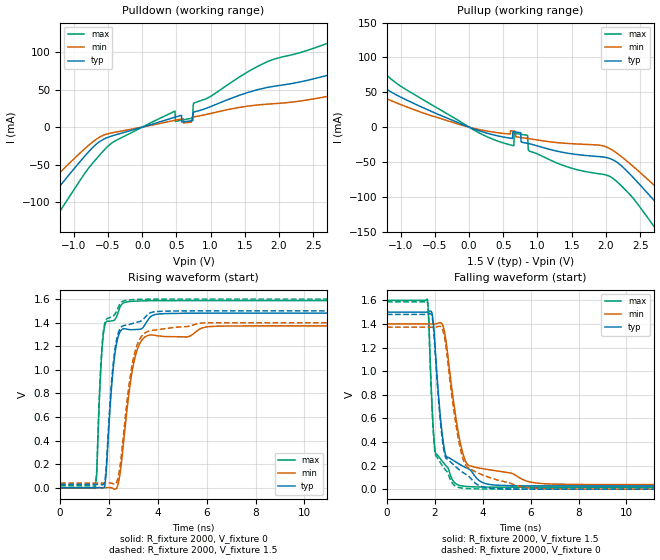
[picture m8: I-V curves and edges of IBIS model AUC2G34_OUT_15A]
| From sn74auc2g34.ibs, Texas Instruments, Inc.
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[Model]   AUC2G34_OUT_15A
Model_type  Output
Vref =   0
Rref =   2000
Cref =   15p
Vmeas =   0.75
| variable   typ   min   max
C_comp   6.42pF   1.69pF   19.07pF
| C_pullup   6.14pF   1.69pF   19.07pF
| C_pulldown   6.71pF   3.61pF   15.24pF
[Temperature Range]   40   100   -40
| Ambient temperature   25   85   -40
[Voltage range]   1.5   1.4   1.6
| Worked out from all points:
|   slope of the pulldown table from 0 to 0.225 V, typ, clamps not added: 36.6 ohm
|   slope of the pullup table from 0 to 0.225 V, typ, clamps not added: 29.5 ohm
|   rising waveform, R_fixture 2000, V_fixture 0: 20-80 % time 344ps typ, 515ps min, 222ps max; typ from 0 V to 1.48 V
|   falling waveform, R_fixture 2000, V_fixture 1.5: 20-80 % time 403ps typ, 614ps min, 233ps max; typ from 1.5 V to 0.027 V
|   rising waveform, R_fixture 2000, V_fixture 1.5: 20-80 % time 338ps typ, 508ps min, 219ps max; typ from 0.027 V to 1.5 V
|   falling waveform, R_fixture 2000, V_fixture 0: 20-80 % time 406ps typ, 619ps min, 231ps max; typ from 1.48 V to 0 V
[Pulldown]
| AUC2G34_OUT_15A
|   Voltage   I(typ)   I(min)   I(max)
-3.6V     -343.5mA   -285.3mA   -424.2mA
-2.1V     -178.7mA   -143.8mA   -232mA
-1.795V   -144.9mA   -115.3mA   -192.2mA
-1.395V   -99.99mA   -78.12mA   -138.8mA
-395mV    -10.45mA   -6.753mA   -18.28mA
480mV     13.33mA    9.224mA    21.44mA
485mV     13.46mA    9.315mA    7.619mA
735mV     8.725mA    13.4mA     12.06mA
755mV     20.22mA    13.7mA     32.02mA
1.69V     50.1mA     29.63mA    81.31mA
3.34V     86.08mA    49.98mA    134.3mA
7.2V      80.61mA    45.5mA     141.2mA
[Pullup]
| AUC2G34_OUT_15A
|   Voltage   I(typ)   I(min)   I(max)
-3.6V     253.3mA    194.5mA    303.7mA
-2.87V    186.5mA    147.2mA    232.6mA
-2.45V    149.4mA    116mA      191.5mA
-1.91V    104.2mA    79.12mA    139.3mA
100mV     -3.652mA   -2.395mA   -5.808mA
650mV     -6.722mA   -5.655mA   -26.6mA
855mV     -23.23mA   -16.19mA   -11.7mA
885mV     -23.9mA    -16.64mA   -34.51mA
2.105V    -46.98mA   -33.57mA   -73.64mA
2.765V    -111.9mA   -88.75mA   -150.9mA
3.365V    -178.9mA   -144.3mA   -231.8mA
7.2V      -606.7mA   -511.1mA   -734.8mA
[Ramp]
| AUC2G34_OUT_15A
| variable   typ   min   max
dV/dt_r   0.89/3.46E-10   0.83/5.21E-10   0.96/2.24E-10
dV/dt_f   0.89/4.05E-10   0.82/6.15E-10   0.96/2.36E-10
R_load = 2000
[Rising Waveform]
| AUC2G34_OUT_15A
R_fixture =   2000
C_fixture =   0
L_fixture =   0
V_fixture =   0
V_fixture_min = 0
V_fixture_max = 0
|   Time   V(typ)   V(min)   V(max)
0s        7.019nV    26.23nV    876.1pV
1.43ns    -7.447uV   -3.74uV    -6.582mV
1.495ns   52.17uV    -6.646uV   114.3mV
1.68ns    -986.3uV   -16.13uV   1.063V
1.82ns    6.054mV    148.5uV    1.368V
2.225ns   1.108V     -12.52mV   1.422V
2.63ns    1.349V     453.2mV    1.57V
3.065ns   1.342V     1.106V     1.583V
3.635ns   1.435V     1.293V     1.586V
22.5ns    1.481V     1.373V     1.587V
[Falling Waveform]
| AUC2G34_OUT_15A
R_fixture =   2000
C_fixture =   0
L_fixture =   0
V_fixture =   1.5
V_fixture_min = 1.4
V_fixture_max = 1.6
|   Time   V(typ)   V(min)   V(max)
0s        1.5V       1.4V       1.6V
1.685ns   1.5V       1.4V       1.609V
1.88ns    1.488V     1.399V     711.4mV
2.015ns   1.181V     1.399V     317mV
2.225ns   618.6mV    1.411V     258.6mV
2.41ns    321.2mV    1.323V     211mV
2.97ns    218.2mV    486.5mV    35.39mV
3.4ns     173.2mV    201.7mV    21.86mV
6.265ns   27.64mV    51.29mV    16.5mV
22.5ns    27.2mV     38.79mV    16.41mV
[Rising Waveform]
| AUC2G34_OUT_15A
R_fixture =   2000
C_fixture =   0
L_fixture =   0
V_fixture =   1.5
V_fixture_min = 1.4
V_fixture_max = 1.6
|   Time   V(typ)   V(min)   V(max)
0s        27.17mV    38.78mV    16.4mV
1.43ns    27.17mV    38.77mV    10.16mV
1.495ns   27.22mV    38.77mV    137.3mV
1.675ns   26.52mV    38.77mV    1.073V
1.82ns    39.89mV    38.92mV    1.388V
2.21ns    1.121V     28.53mV    1.464V
2.6ns     1.375V     463.9mV    1.584V
3.06ns    1.399V     1.151V     1.596V
3.71ns    1.485V     1.332V     1.599V
22.5ns    1.5V       1.4V       1.6V
[Falling Waveform]
| AUC2G34_OUT_15A
R_fixture =   2000
C_fixture =   0
L_fixture =   0
V_fixture =   0
V_fixture_min = 0
V_fixture_max = 0
|   Time   V(typ)   V(min)   V(max)
0s        1.481V     1.373V     1.587V
1.685ns   1.481V     1.373V     1.594V
1.875ns   1.468V     1.372V     706.8mV
2.015ns   1.143V     1.372V     297.3mV
2.22ns    591.8mV    1.38V      228.3mV
2.395ns   308.3mV    1.293V     175mV
2.95ns    175.6mV    457mV      17.41mV
3.35ns    118.6mV    185.2mV    5.603mV
5.87ns    612.6uV    11.95mV    119.8uV
22.5ns    28.2uV     4.814uV    11.67uV
